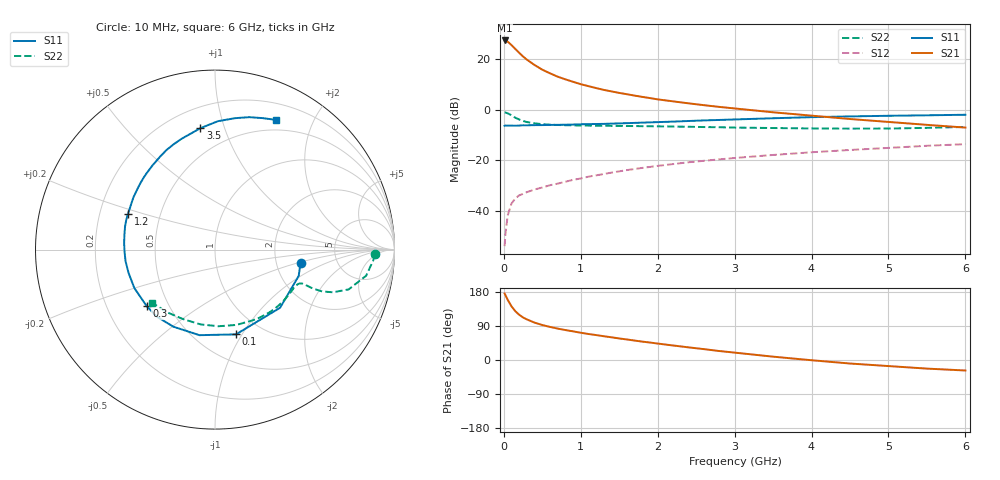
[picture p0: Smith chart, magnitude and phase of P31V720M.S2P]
! SIEMENS Small Signal Semiconductors
! BFP181
! Si NPN RF Bipolar Junction Transistor in SOT143
! VCE = 1.75 V  IC = 20 mA
! Common Emitter S-Parameters:  March  1996
# GHz  S  MA  R  50
!  f  S11  S21  S12  S22
! GHz  MAG  ANG  MAG  ANG  MAG  ANG  MAG  ANG
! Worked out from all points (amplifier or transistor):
!   36 points, 10 MHz to 6 GHz, reference 50 ohm
!   highest |S21| = 27.5 dB at 10 MHz (marker M1)
!   |S21| within 3 dB of that: start of sweep to 137.3 MHz
!   unconditionally stable (mu >= 1): start of sweep to 23.3 MHz; 296.3 MHz to end of sweep
!   at 250 MHz: K = 0.90, MSG = 27.2 dB, |S12| = -33.3 dB
!   at 1.4 GHz: K = 1.89, MAG = 10.6 dB, |S12| = -24.9 dB
!   at 6 GHz: K = 1.46, MAG = -0.7 dB, |S12| = -13.6 dB
!   S11 on the Smith chart (normalised r, x): 10 MHz: 2.74, -0.55; 100 MHz: 0.76, -0.94; 300 MHz: 0.38, -0.31; 1.2 GHz: 0.32, +0.18; 3.5 GHz: 0.33, +0.83; 6 GHz: 0.38, +1.51
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0.01  0.4826 -9.1  23.62 175.6  0.002 72.4  0.8893 -1.7
0.02  0.4888 -17.5  23.55 171.5  0.0034 72.1  0.8839 -3.9
0.05  0.4863 -41.8  22.39 158.8  0.0081 74.3  0.8546 -9.8
0.1  0.4866 -76.1  19.09 141.5  0.014 60.5  0.7768 -16.6
0.15  0.4846 -100.3  15.98 128.6  0.0177 54.3  0.6983 -19.9
0.2  0.4881 -118.3  13.43 119.3  0.0203 50.1  0.6425 -21.3
0.25  0.4947 -131.0  11.36 112.2  0.0217 47.8  0.6006 -21.6
0.3  0.4939 -140.5  9.844 107.1  0.0235 47.0  0.5735 -21.6
0.4  0.4979 -154.5  7.699 98.6  0.0265 47.9  0.5394 -21.3
0.5  0.4989 -164.9  6.232 92.3  0.029 48.9  0.5206 -21.3
0.6  0.5026 -172.7  5.282 87.3  0.0322 50.2  0.5082 -21.8
0.7  0.5043 -178.9  4.53 82.9  0.0346 52.1  0.501 -22.5
0.8  0.5076 175.9  4.013 79.0  0.0377 53.6  0.4964 -23.4
1.1  0.5215 161.4  2.942 68.6  0.0475 55.5  0.4868 -27.0
1.2  0.5241 157.8  2.694 65.8  0.0505 55.6  0.485 -28.5
1.7  0.5514 140.7  1.912 51.3  0.0675 55.7  0.4768 -36.6
2.2  0.5844 126.5  1.472 38.3  0.0844 53.7  0.4666 -45.8
2.8  0.6302 111.5  1.143 23.7  0.1045 50.0  0.4522 -58.2
3.5  0.6812 96.9  0.894 8.8  0.1278 45.0  0.4362 -74.2
4.5  0.7408 81.3  0.658 -9.3  0.1605 36.6  0.4245 -100.8
5.5  0.7791 70.1  0.504 -22.7  0.1942 28.0  0.4397 -127.4
6  0.7988 64.8  0.445 -27.7  0.2092 23.1  0.4587 -139.9
